TYPE SPLC_TO_PLC :
STRUCT
	EV1_EN,
	EV2_EN,
	EV3_EN,
	EV4_EN,
	HTR_APC_EN,
	HTR_CHAMBER_EN,
	HTR_FORLINE_EN,
	HTR_GAS_BOX,
	HTR_GATE_VALVE,
	HTR_LID,
	PROCESS_EN,
	DRY_PUMP_PW_EN,
	TMP_PW_EN,
	TRANSFER_EN,
	VALVE_ACID_EXHAUST_OPEN_EN,
	VALVE_CM_OPEN_EN,	
	VALVE_DRY_PUMP_EN,
	VALVE_TMP_BACK_OPEN_EN,
	VALVE_APC_OPEN_EN,
	WAFER_MOVING_IN_EN,	
	Status_Lid	,
	SPLC_Com_err,
	SPLC_FB_Err,
	Other_Err 	 	:BOOL;
END_STRUCT
END_TYPE
